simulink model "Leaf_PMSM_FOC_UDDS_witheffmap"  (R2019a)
settings: Solver=VariableStepAuto  StartTime=0.0  StopTime=764  FixedStep=1e-3  MaxStep=1e-3  RelTol=1e-3
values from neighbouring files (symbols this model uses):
  B = 0    [PMSM_EV_init_v2.m]    (also in Leaf_Initialization.m; Tesla_Initialization.m)
  Eoff = 201e-6    (= 0.000201)    [DeviceParam.m]
  Eoff_diode = 1.4e-3    (= 0.0014)    [DeviceParam.m]
  Eoff_Si = 2.15e-3    (= 0.00215)    [DeviceParam.m]
  Eon = 252e-6    (= 0.000252)    [DeviceParam.m]
  Eon_Si = 1.2e-3    (= 0.0012)    [DeviceParam.m]
  fs = 10000    [PMSM_EV_init_v2.m]    (also in Leaf_Initialization.m; Tesla_Initialization.m)
  I_DS_data = [-36 36 62]    [DeviceParam.m]
  IC_data = [0 30 60]    [DeviceParam.m]
  Inom = 75    [DeviceParam.m]    (also in Iqbal Husain - Example12_1.m = Psm/VsmNom)
  J = 0.3    [PMSM_EV_init_v2.m]    (also in Leaf_Initialization.m; Tesla_Initialization.m)
  Leaf_id_axis = [-2.296328E+02	-2.041181E+02	-1.786033E+02	-1.530886E+02	-1.275738E+02	-1.020590E+02	-7.654428E+01	-5.102952E+01	-2.551476E+01	+0.000000E+00]    [Leaf_Param.m]    (also in Leaf_Initialization.m)
  Leaf_iq_axis = [+0.000000E+00	+2.551476E+01	+5.102952E+01	+7.654428E+01	+1.020590E+02	+1.275738E+02	+1.530886E+02	+1.786033E+02	+2.041181E+02	+2.296328E+02]    [Leaf_Param.m]    (also in Leaf_Initialization.m)
  Leaf_Ld = [+4.562516E-04	+4.676675E-04	+4.893199E-04	+5.037353E-04	+5.104223E-04	+5.166612E-04	+5.237499E-04	+5.295159E-04	+5.345150E-04	+5.371060E-04    [Leaf_Param.m]    (also in Leaf_Initialization.m)
  Leaf_Lq = [+1.028048E-03	+1.047482E-03	+1.072792E-03	+1.100303E-03	+1.125549E-03	+1.152180E-03	+1.181188E-03	+1.211466E-03	+1.243133E-03	+1.273628E-03    [Leaf_Param.m]    (also in Leaf_Initialization.m)
  Leaf_omega_axis = [+0.000000E+00	+3.935365E+01	+7.870730E+01	+1.180610E+02	+1.574146E+02	+1.967683E+02	+2.361219E+02	+2.754756E+02	+3.857216E+02	+4.959676E+02	+6.062136E+02	+7.164596E+02	+8.267056E+02	+9.369516E+02	+1.047198E+03]    [Leaf_Param.m]    (also in Leaf_Initialization.m)
  Leaf_phid = [-4.199708E-02	-2.553401E-02	-8.247090E-03	+9.778563E-03	+2.810579E-02	+4.661402E-02	+6.539149E-02	+8.441129E-02	+1.036049E-01	+1.229854E-01    [Leaf_Param.m]    (also in Leaf_Initialization.m)
  Leaf_phiq = [-1.952292E-05	-3.396145E-06	+2.962394E-07	-2.077424E-05	-3.654397E-05	-1.649631E-05	+3.339687E-05	+4.306712E-05	+9.669480E-06	-2.373166E-05    [Leaf_Param.m]    (also in Leaf_Initialization.m)
  Leaf_T = [-3.804040E-02	-5.882121E-03	+4.489506E-04	-2.698573E-02	-3.955883E-02	-1.428580E-02	+2.169126E-02	+1.864805E-02	+2.093441E-03	+0.000000E+00    [Leaf_Param.m]    (also in Leaf_Initialization.m)
  Leaf_torque_axis = [+0.000000E+00	+1.167089E+01	+2.334179E+01	+3.501268E+01	+4.668357E+01	+5.835446E+01	+7.002536E+01	+7.910792E+01	+9.076234E+01	+1.063042E+02	+1.281510E+02	+1.612785E+02	+2.121831E+02	+2.805757E+02]    [Leaf_Param.m]    (also in Leaf_Initialization.m)
  P = 8    [PMSM_EV_init_v2.m]    (also in Iqbal Husain - Example12_1.m = V.*I; Leaf_Initialization.m; Tesla_Initialization.m)
  Rd_IGBT = (1.4-0.9)/(60-15)    (= 0.0111111111111)    [DeviceParam.m]
  RDS_on_data = [25e-3 27e-3 28e-3]    [DeviceParam.m]
  Rs = 0.046    [PMSM_EV_init_v2.m]    (also in Leaf_Initialization.m; Tesla_Initialization.m)
  Speed = [+0.000000E+00	+6.054730E+02	+1.210946E+03	+1.816419E+03	+2.421892E+03	+3.027365E+03	+3.632838E+03	+4.238311E+03	+5.775695E+03	+7.313079E+03	+8.850463E+03	+1.038785E+04	+1.192523E+04	+1.346262E+04	+1.500000E+04]    [PMSM_EV_init_v2.m]
  Torque = [+0.000000E+00	+7.333624E+00	+1.466725E+01	+2.200087E+01	+2.933450E+01	+3.666812E+01	+4.400174E+01	+5.043561E+01	+5.870849E+01	+6.980054E+01	+8.566293E+01	+1.107686E+02	+1.535327E+02	+2.089386E+02]    [PMSM_EV_init_v2.m]
  Vbatt = Vdc    (= 375)    [PMSM_EV_init_v2.m]    (also in Leaf_Initialization.m; Tesla_Initialization.m)
  VCE_data = [0 1.1 1.45]    [DeviceParam.m]
  Vd_IGBT = 1.5    [DeviceParam.m]
  Vdc = 375    [PMSM_EV_init_v2.m]    (also in Leaf_Initialization.m; Tesla_Initialization.m)
  Vnom = 300    [DeviceParam.m]
undefined symbols (not defined in the file or in its folder): A1, B1370, B766, HEV_Param, plecs
libraries: fl_lib x18, nesl_utility x9, sdl_lib x4, powerlib_meascontrol x3
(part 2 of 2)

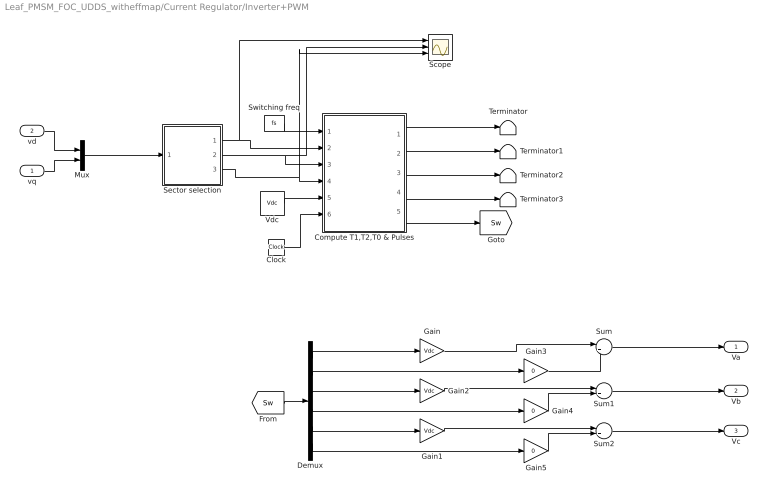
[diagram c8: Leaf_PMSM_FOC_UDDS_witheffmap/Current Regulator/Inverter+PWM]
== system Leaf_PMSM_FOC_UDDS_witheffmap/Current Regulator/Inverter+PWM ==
  vq : Inport
  vd : Inport  Port=2
  Clock : Clock
  Compute T1,T2,T0 & Pulses : MATLAB Function  TreatAsAtomicUnit=on
  Demux : Demux  Outputs=6
  Gain : Gain  Gain=Vdc
  Gain1 : Gain  Gain=Vdc
  Gain2 : Gain  Gain=Vdc
  Gain3 : Gain  Gain=0
  Gain4 : Gain  Gain=0
  Gain5 : Gain  Gain=0
  Mux : Mux  Inputs=2
  Scope : Scope  NumInputPorts=3
  Sector selection : MATLAB Function  TreatAsAtomicUnit=on
  Sum : Sum  Inputs=|++
  Sum1 : Sum  Inputs=|++
  Sum2 : Sum  Inputs=|++
  Switching freq : Constant  Value=fs
  Terminator{,1..3} (4 alike) : Terminator
  Vdc : Constant  Value=Vdc
  Va : Outport
  Vb : Outport  Port=2
  Vc : Outport  Port=3
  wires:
  Compute T1,T2,T0 & Pulses/1(T1) -> Terminator/1
  Compute T1,T2,T0 & Pulses/2(T2) -> Terminator1/1
  vq/1 -> Mux/2
  Vdc/1 -> Compute T1,T2,T0 & Pulses/5(Vdc)
  Mux/1 -> Sector selection/1(u)
  Sector selection/1(Mag) -> Scope/1, Compute T1,T2,T0 & Pulses/2(Mag)
  Compute T1,T2,T0 & Pulses/3(T0) -> Terminator2/1
  Sector selection/3(Sec) -> Scope/3, Compute T1,T2,T0 & Pulses/4(Sec)
  Sector selection/2(ang) -> Scope/2, Compute T1,T2,T0 & Pulses/3(ang)
  [Sw] -> Demux/1
  vd/1 -> Mux/1
  Switching freq/1 -> Compute T1,T2,T0 & Pulses/1(Fs)
  Compute T1,T2,T0 & Pulses/5(Pulse) -> [Sw]
  Clock/1 -> Compute T1,T2,T0 & Pulses/6(clk)
  Compute T1,T2,T0 & Pulses/4(Time_int) -> Terminator3/1
  Demux/1 -> Gain/1
  Demux/3 -> Gain2/1
  Demux/5 -> Gain1/1
  Demux/2 -> Gain3/1
  Demux/6 -> Gain5/1
  Demux/4 -> Gain4/1
  Gain/1 -> Sum/1
  Gain3/1 -> Sum/2
  Gain2/1 -> Sum1/1
  Gain4/1 -> Sum1/2
  Gain1/1 -> Sum2/1
  Gain5/1 -> Sum2/2
  Sum/1 -> Va/1
  Sum1/1 -> Vb/1
  Sum2/1 -> Vc/1

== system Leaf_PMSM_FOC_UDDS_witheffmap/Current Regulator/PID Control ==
  In1 : Inport
  In3 : Inport  Port=2
  Gain : Gain  Gain=10
  Gain1 : Gain  Gain=10
  Gain2 : Gain
  Gain3 : Gain
  Integrator : Integrator
  Integrator1 : Integrator
  Scope : Scope  NumInputPorts=2
  Sum2 : Sum  Inputs=|++
  Sum3 : Sum  Inputs=|++
  Out1 : Outport
  Out2 : Outport  Port=2
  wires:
  Integrator1/1 -> Gain3/1
  Gain1/1 -> Scope/2, Sum3/1
  Gain2/1 -> Sum2/2
  Gain/1 -> Scope/1, Sum2/1
  In1/1 -> Integrator/1, Gain/1
  Sum2/1 -> Out1/1
  In3/1 -> Integrator1/1, Gain1/1
  Integrator/1 -> Gain2/1
  Gain3/1 -> Sum3/2
  Sum3/1 -> Out2/1

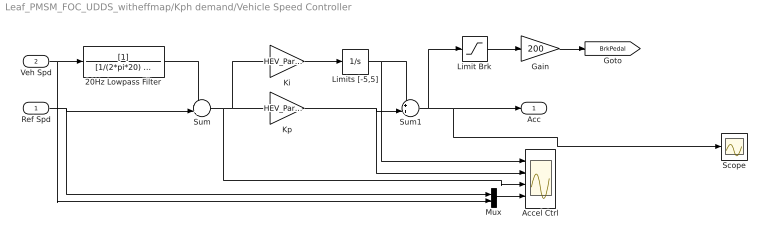
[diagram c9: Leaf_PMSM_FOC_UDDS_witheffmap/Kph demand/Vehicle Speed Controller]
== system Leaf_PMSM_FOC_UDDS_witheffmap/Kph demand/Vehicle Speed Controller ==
  Ref Spd : Inport
  Veh Spd : Inport  Port=2
  20Hz Lowpass Filter : TransferFcn  Denominator=[1/(2*pi*20) 1]
  Accel Ctrl : Scope  NumInputPorts=4
  Gain : Gain  Gain=200
  Ki : Gain  Gain=HEV_Param.Control.Veh_Spd.Ki
  Kp : Gain  Gain=HEV_Param.Control.Veh_Spd.Kp
  Limit Brk : Saturate  UpperLimit=0  LowerLimit=-inf
  Limits [-5,5] : Integrator  LimitOutput=on  UpperSaturationLimit=8  LowerSaturationLimit=-8
  Mux : Mux  Inputs=2
  Scope : Scope
  Sum : Sum  Inputs=-+|
  Sum1 : Sum  Inputs=++|
  Acc : Outport
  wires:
  Ref Spd/1 -> Sum/2, Mux/1
  Veh Spd/1 -> 20Hz Lowpass Filter/1, Mux/2
  Sum/1 -> Ki/1, Kp/1, Accel Ctrl/3
  Ki/1 -> Limits [-5,5]/1
  Kp/1 -> Accel Ctrl/2, Sum1/2
  Limits [-5,5]/1 -> Accel Ctrl/1, Sum1/1
  20Hz Lowpass Filter/1 -> Sum/1
  Mux/1 -> Accel Ctrl/4
  Limit Brk/1 -> Gain/1
  Gain/1 -> [BrkPedal]
  Sum1/1 -> Scope/1, Acc/1, Limit Brk/1

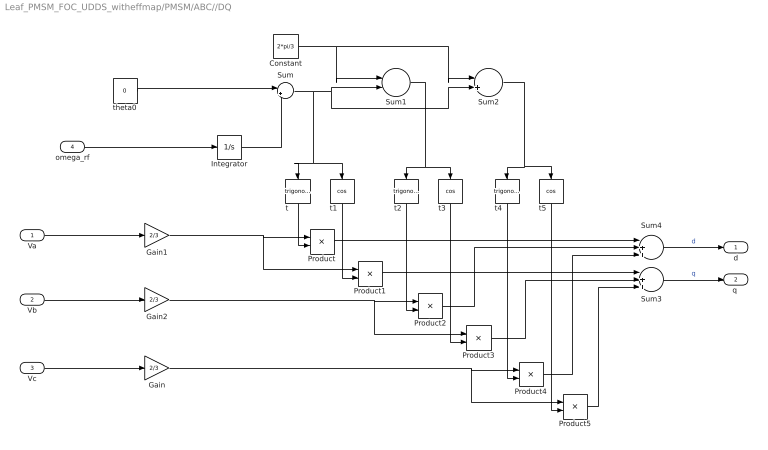
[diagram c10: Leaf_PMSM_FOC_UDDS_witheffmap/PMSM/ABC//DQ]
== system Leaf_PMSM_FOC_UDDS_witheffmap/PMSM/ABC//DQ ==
  Va : Inport
  Vb : Inport  Port=2
  Vc : Inport  Port=3
  omega_rf : Inport  Port=4
  Constant : Constant  Value=2*pi/3
  Gain : Gain  Gain=2/3
  Gain1 : Gain  Gain=2/3
  Gain2 : Gain  Gain=2/3
  Integrator : Integrator
  Product{,1..5} (6 alike) : Product
  Sum : Sum  Inputs=|++
  Sum1 : Sum  Inputs=|-+
  Sum2 : Sum  Inputs=|++
  Sum3 : Sum  Inputs=|+++
  Sum4 : Sum  Inputs=|+++
  t : Trigonometry
  t1 : Trigonometry  Operator=cos
  t2 : Trigonometry
  t3 : Trigonometry  Operator=cos
  t4 : Trigonometry
  t5 : Trigonometry  Operator=cos
  theta0 : Constant  Value=0
  d : Outport
  "q " : Outport  Port=2
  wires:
  theta0/1 -> Sum/1
  Sum/1 -> t1/1, t/1, Sum2/2, Sum1/2
  Sum2/1 -> t5/1, t4/1
  Integrator/1 -> Sum/2
  t4/1 -> Product4/2
  Sum1/1 -> t2/1, t3/1
  Product/1 -> Sum4/1
  t/1 -> Product/2
  Va/1 -> Gain1/1
  Constant/1 -> Sum1/1, Sum2/1
  Vc/1 -> Gain/1
  Product3/1 -> Sum3/2
  Gain2/1 -> Product3/1, Product2/1
  t5/1 -> Product5/2
  t1/1 -> Product1/2
  Gain/1 -> Product5/1, Product4/1
  Product1/1 -> Sum3/1
  Gain1/1 -> Product1/1, Product/1
  Product5/1 -> Sum3/3
  Product2/1 -> Sum4/2
  Product4/1 -> Sum4/3
  Vb/1 -> Gain2/1
  t3/1 -> Product3/2
  t2/1 -> Product2/2
  Sum4/1 -> d/1  "d"
  Sum3/1 -> "q "/1  "q"
  omega_rf/1 -> Integrator/1

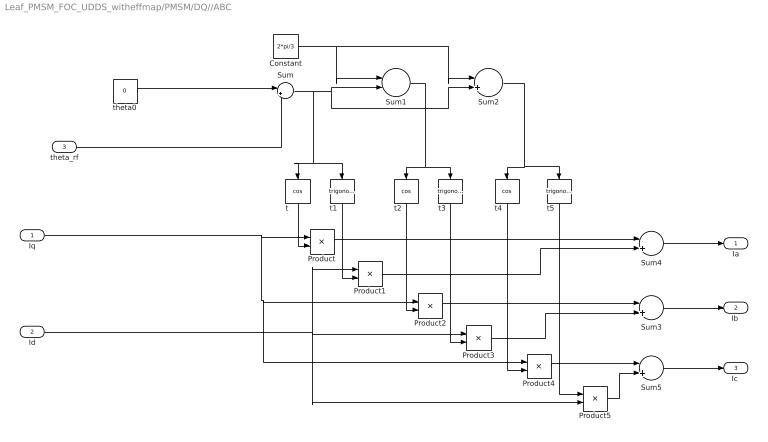
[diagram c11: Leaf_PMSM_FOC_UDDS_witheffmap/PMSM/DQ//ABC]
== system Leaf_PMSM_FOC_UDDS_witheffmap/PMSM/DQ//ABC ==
  Iq : Inport
  Id : Inport  Port=2
  theta_rf : Inport  Port=3
  Constant : Constant  Value=2*pi/3
  Product{,1..5} (6 alike) : Product
  Sum{,2..5} (5 alike) : Sum  Inputs=|++
  Sum1 : Sum  Inputs=|-+
  t : Trigonometry  Operator=cos
  t1 : Trigonometry
  t2 : Trigonometry  Operator=cos
  t3 : Trigonometry
  t4 : Trigonometry  Operator=cos
  t5 : Trigonometry
  theta0 : Constant  Value=0
  Ia : Outport
  "Ib " : Outport  Port=2
  "Ic " : Outport  Port=3
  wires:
  theta0/1 -> Sum/1
  Sum/1 -> t1/1, t/1, Sum2/2, Sum1/2
  Sum2/1 -> t5/1, t4/1
  Sum1/1 -> t2/1, t3/1
  t/1 -> Product/2
  Constant/1 -> Sum1/1, Sum2/1
  Product3/1 -> Sum3/2
  t1/1 -> Product1/2
  t3/1 -> Product3/2
  t2/1 -> Product2/2
  Sum4/1 -> Ia/1
  Sum3/1 -> "Ib "/1
  theta_rf/1 -> Sum/2
  Id/1 -> Product5/2, Product1/1, Product3/1
  Product/1 -> Sum4/1
  Product1/1 -> Sum4/2
  Product2/1 -> Sum3/1
  Iq/1 -> Product4/1, Product2/1, Product/1
  t4/1 -> Product4/2
  t5/1 -> Product5/1
  Product4/1 -> Sum5/1
  Product5/1 -> Sum5/2
  Sum5/1 -> "Ic "/1

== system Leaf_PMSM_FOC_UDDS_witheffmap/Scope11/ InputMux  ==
  In1 : Inport
  Convert1 : DataTypeConversion
  Mux : Mux  Inputs=1
  Out : Outport
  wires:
  Mux/1 -> Out/1
  In1/1 -> Convert1/1
  Convert1/1 -> Mux/1

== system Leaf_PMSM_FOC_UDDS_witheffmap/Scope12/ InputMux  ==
  In1 : Inport
  Convert1 : DataTypeConversion
  Mux : Mux  Inputs=1
  Out : Outport
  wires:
  Mux/1 -> Out/1
  In1/1 -> Convert1/1
  Convert1/1 -> Mux/1

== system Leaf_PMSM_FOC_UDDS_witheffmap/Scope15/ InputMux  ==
  In1 : Inport
  Convert1 : DataTypeConversion
  Mux : Mux  Inputs=1
  Out : Outport
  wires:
  Mux/1 -> Out/1
  In1/1 -> Convert1/1
  Convert1/1 -> Mux/1

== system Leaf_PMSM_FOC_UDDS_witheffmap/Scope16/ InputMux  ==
  In1 : Inport
  Convert1 : DataTypeConversion
  Mux : Mux  Inputs=1
  Out : Outport
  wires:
  Convert1/1 -> Mux/1
  In1/1 -> Convert1/1
  Mux/1 -> Out/1

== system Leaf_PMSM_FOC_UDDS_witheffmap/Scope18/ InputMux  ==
  In1 : Inport
  Convert1 : DataTypeConversion
  Mux : Mux  Inputs=1
  Out : Outport
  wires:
  Mux/1 -> Out/1
  In1/1 -> Convert1/1
  Convert1/1 -> Mux/1

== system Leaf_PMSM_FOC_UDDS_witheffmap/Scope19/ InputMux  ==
  In1 : Inport
  Convert1 : DataTypeConversion
  Mux : Mux  Inputs=1
  Out : Outport
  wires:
  Convert1/1 -> Mux/1
  In1/1 -> Convert1/1
  Mux/1 -> Out/1

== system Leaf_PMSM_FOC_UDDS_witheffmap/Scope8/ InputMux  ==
  In1 : Inport
  Convert1 : DataTypeConversion
  Mux : Mux  Inputs=1
  Out : Outport
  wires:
  Convert1/1 -> Mux/1
  In1/1 -> Convert1/1
  Mux/1 -> Out/1

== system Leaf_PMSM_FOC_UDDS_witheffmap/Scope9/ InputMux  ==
  In1 : Inport
  Convert1 : DataTypeConversion
  Mux : Mux  Inputs=1
  Out : Outport
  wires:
  Convert1/1 -> Mux/1
  In1/1 -> Convert1/1
  Mux/1 -> Out/1

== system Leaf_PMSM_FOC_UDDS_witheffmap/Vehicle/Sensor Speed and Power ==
  Ideal Rotational Motion Sensor : fl_lib/Mechanical/Mechanical Sensors/Ideal Rotational Motion Sensor  offset=0 rad
  Ideal Torque Sensor : fl_lib/Mechanical/Mechanical Sensors/Ideal Torque Sensor
  Mechanical Rotational Reference : fl_lib/Mechanical/Rotational Elements/Mechanical Rotational Reference
  PS-Simulink Converter : nesl_utility/PS-Simulink Converter  PhysicalDomain=network_engine_domain  SubClassName=ps_output  LeftPortType=input  RightPortType=output  PseudoPeriodic=off  Frequencies=[]  Unit=N*m  AffineConversion=off
  PS-Simulink Converter1 : nesl_utility/PS-Simulink Converter  PhysicalDomain=network_engine_domain  SubClassName=ps_output  LeftPortType=input  RightPortType=output  PseudoPeriodic=off  Frequencies=[]  Unit=rad/s  AffineConversion=off
  Product : Product
  W2kW : Gain  Gain=0.001
  B : PMIOPort  Side=Left
  F : PMIOPort  Port=2  Side=Right
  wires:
  W2kW/1 -> [Pm_vehicle]
  Product/1 -> W2kW/1
  PS-Simulink Converter/1 -> Product/1
  PS-Simulink Converter1/1 -> Product/2
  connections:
  Mechanical Rotational Reference/LConn1 -- Ideal Rotational Motion Sensor/RConn1
  Ideal Rotational Motion Sensor/LConn1 -- F/RConn1 -- Ideal Torque Sensor/RConn1
  B/RConn1 -- Ideal Torque Sensor/LConn1
  PS-Simulink Converter/LConn1 -- Ideal Torque Sensor/RConn2
  PS-Simulink Converter1/LConn1 -- Ideal Rotational Motion Sensor/RConn2

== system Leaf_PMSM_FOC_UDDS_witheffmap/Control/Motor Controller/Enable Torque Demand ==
  Mot_Enable : Inport
  TrqDemCtrl : Inport  Port=2
  20Hz Lowpass Filter : TransferFcn  Denominator=[1/(2*pi*10) 1]
  Product : Product
  Scope : Scope
  Select Logic : ManualSwitch  CurrentSetting=0
  TrqDem : Outport
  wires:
  Mot_Enable/1 -> 20Hz Lowpass Filter/1
  TrqDemCtrl/1 -> Product/2, Select Logic/2
  Product/1 -> Select Logic/1
  20Hz Lowpass Filter/1 -> Product/1
  Select Logic/1 -> Scope/1, TrqDem/1

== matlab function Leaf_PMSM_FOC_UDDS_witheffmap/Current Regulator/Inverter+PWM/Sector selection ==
function [Mag,ang,Sec] = fcn(u)
%convert to polar format
z=u(1)+ i* u(2);
Mag=abs(z);
ang=atan2(imag(z),real(z));
alpha=ang*180/pi;

% Sector calculation
Sec = (alpha>0 & alpha<=60)*1+ (alpha>60 & alpha<=120)*2  + (alpha>120 & alpha<=180)*3 ...
  +(alpha>-180 & alpha<-120)*4+ (alpha>-120 & alpha<=-60)*5 + (alpha>-60 & alpha<=0)*6;


%  determine whether sector is an odd number
% odd_sec=mod(floor(Sec),2);

== matlab function Leaf_PMSM_FOC_UDDS_witheffmap/Current Regulator/Inverter+PWM/Compute T1,T2,T0
& Pulses ==
function [T1,T2,T0,Time_int,Pulse] = fcn(Fs,Mag,ang,Sec,Vdc,clk)
% synchronise simulation time with simulink
t=clk;

 %Vdc from simulink workspace
% Compute Times for segments
m=sqrt(3)*(Mag/Vdc);
T1=m*sin(Sec*pi/3 -ang)/Fs;
T2=m*sin(ang - ((Sec-1)*pi/3))/Fs;
T0= (1/Fs -T1- T2)/2;

% Determin whether odd sector. (to swap the oder of vector placement) 
% ie for odd sector T1,T2, To  and for even sector T2,T1,T0
 odd_sec=mod(floor(Sec),2);
if(odd_sec~=1)  %ie an even sector%
 T1=m*sin(ang - ((Sec-1)*pi/3))/Fs;
 T2=m*sin(Sec*pi/3 -ang)/Fs;
end


% sawtooth signal
ref= 1/Fs * rem(t,1/Fs)/(1/Fs);


% sub interval timings
int1=T0/4;
int2=int1+T1/2;
int3=int2+T2/2;
int4=int3+T0/2;
int5=int4+T2/2;
int6=int5+T1/2;

Time_int=1+(ref>=int1)+(ref>=int2)+(ref>=int3)+(ref>=int4)+(ref>=int5)+(ref>=int6);
% 
% % format of the array sw_array(x,y,z)
sw_array=zeros(3,7,6);  % initialize the switching table
% % x=[legA Leg B LegC] % y=[Timeint1 timeint2 ..] % Z=[sector1 sector2 ..]
sw_array(:,:,1)=[0	1	1	1	1	1	0;0  0	1	1	1	0	0; 0	0	0	1	0	0	0]; %sector 1
sw_array(:,:,2)=[0	0	1	1	1	0	0;0	 1	1	1	1	1	0; 0	0	0	1	0	0	0]; %sector 2
sw_array(:,:,3)=[0	0	0	1	0	0	0;0	 1	1	1	1	1	0; 0	0	1	1	1	0	0]; %sector 3
sw_array(:,:,4)=[0	0	0	1	0	0	0;0	 0	1	1	1	0	0; 0	1	1	1	1	1	0]; %sector 4
sw_array(:,:,5)=[0	0	1	1	1	0	0;0	 0	0	1	0	0	0; 0	1	1	1	1	1	0]; %sector 5
sw_array(:,:,6)=[0	1	1	1	1	1	0;0	 0	0	1	0	0	0; 0	0	1	1	1	0	0]; %sector 6
 

% Adding time delay to allow parameter initialization
if t<50e-6
Sec=1;
end;

S1=sw_array(1,Time_int,Sec);
S2= ~S1;
S3=sw_array(2,Time_int,Sec);
S4= ~S3;
S5=sw_array(3,Time_int,Sec);
S6= ~S5;
% Merged Pulse
Pulse= [S1 S2 S3 S4 S5 S6]';





end
